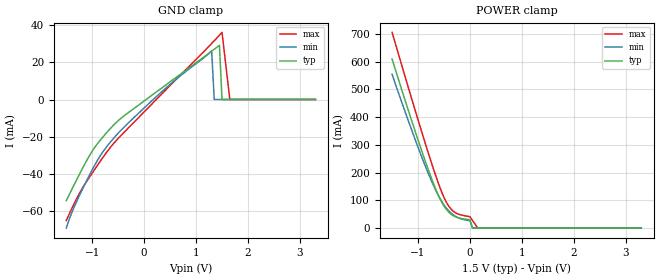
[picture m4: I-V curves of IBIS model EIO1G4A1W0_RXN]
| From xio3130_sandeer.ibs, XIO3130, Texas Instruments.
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|   Model EIO1G4A1W0_RXN
[Model]   EIO1G4A1W0_RXN
Model_type   Input
Polarity   Inverting
Vinl =  -0.6000V
Vinh =   0.6000V
C_comp   1.6030pF   1.5940pF   1.6370pF
[Temperature Range]   25.0000   0.1250k   -40.0000
[Voltage Range]   1.5000V   1.3500V   1.6500V
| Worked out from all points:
|   GND clamp passes 1 mA (typ) near -0.01 V on its own axis
[GND_clamp]
| voltage   I(typ)   I(min)   I(max)
-1.5V     -54.49mA   -69.31mA   -65.2mA
-1.35V    -46.02mA   -58.08mA   -56.26mA
-1.15V    -35.12mA   -46.11mA   -45.96mA
-750mV    -18.74mA   -26.49mA   -29.48mA
-450mV    -10.21mA   -16.64mA   -19.49mA
650mV     12.61mA    11.71mA    11.77mA
1.3V      26.01mA    26.23mA    30.18mA
1.35V     27.05mA    0A         31.65mA
1.45V     29.17mA    0A         34.64mA
1.5V      0A         0A         36.17mA
1.65V     0A         0A         0A
3.3V      0A         0A         0A
[POWER_clamp]
| voltage   I(typ)   I(min)   I(max)
-1.5V     609.3mA    554.5mA    705.7mA
-1.05V    345.9mA    316.4mA    421.1mA
-850mV    235.6mA    218.9mA    299mA
-700mV    159.3mA    152.8mA    211.5mA
-600mV    114.7mA    114.5mA    157.4mA
-500mV    79.46mA    83.42mA    110.5mA
-400mV    56.03mA    60.63mA    76.75mA
-300mV    42.47mA    45.18mA    57.85mA
0V        30.28mA    26.63mA    41.02mA
50mV      0A         0A         27.35mA
150mV     0A         0A         0A
3.3V      0A         0A         0A
